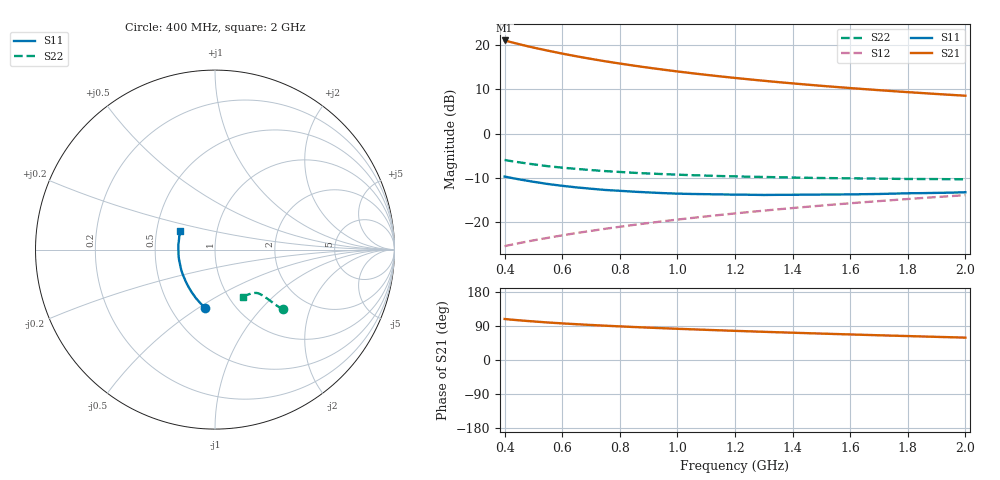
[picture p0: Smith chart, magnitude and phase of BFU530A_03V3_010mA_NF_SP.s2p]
! Filename:  P:\Prog\Test\Noise\ATS_data\Testdata_Net\06 Compressed Noise after Statistics\BFU530A_APG2013_33_A05_03p3V_010mA_NF_CM01_D.sf
! Date/Time: Tue 16/Apr/2013 15:10:58
! BFU530A_APG2013_33_A05_03p3V_1to25mA_NF_CM01_Bias5_R.sf
! Noise Parameter Data File
! BFU530A_APG2013_33_A05_03p3V_1to25mA_NF_CM01
! Date/time: Fri Apr 12 14:21:19 2013
! VAR V_out= 3.300000
! VAR I_out= 10.010000
! VAR V_in= 0.838100
! VAR I_in= 0.109800
! Device data file deembeded for feedlines and parallel
! Original file: \06 Compressed Noise after Statistics\BFU530A_APG2013_33_A05_03p3V_010mA_NF_CM01_R.sf
! Feed-files: PR017V01_150413_Feed1.s2p, PR017V01_150413_Feed2.s2p
! Parallel-file: PR017V01_150413_Par.s2p
# MHz S MA R 50
!  Freq-MHz  S11-mag  S11-arg  S21-mag  S21-arg  S12-mag  S12-arg  S22-mag  S22-arg
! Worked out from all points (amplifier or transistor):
!   37 points, 400 MHz to 2 GHz, reference 50 ohm
!   highest |S21| = 21.0 dB at 400 MHz (marker M1)
!   |S21| within 3 dB of that: start of sweep to 602.7 MHz
!   unconditionally stable (mu >= 1): 1.258 GHz to end of sweep
!   at 500 MHz: K = 0.81, MSG = 21.8 dB, |S12| = -24.1 dB
!   at 1.1 GHz: K = 0.99, MSG = 16.0 dB, |S12| = -18.7 dB
!   at 2 GHz: K = 1.01, MAG = 10.7 dB, |S12| = -13.9 dB
!   lowest NFmin = 0.79 dB at 433 MHz
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400  0.3283 -99.7  11.28 108.2  0.0538 64.5  0.5051 -41.3
420  0.3191 -102.5  10.85 106.7  0.05557 64.6  0.4923 -41.6
440  0.3097 -105.2  10.44 105.4  0.05731 64.7  0.481 -41.8
460  0.3016 -107.7  10.06 104.1  0.05907 64.8  0.4707 -42.1
500  0.2867 -112.7  9.376 101.8  0.06254 65.1  0.4513 -42.4
550  0.2708 -118.6  8.655 99.0  0.06678 65.5  0.4298 -42.7
600  0.2581 -123.9  8.015 96.6  0.07124 65.8  0.4138 -42.9
650  0.2478 -128.8  7.466 94.5  0.07567 66.1  0.4004 -43.2
700  0.2393 -133.6  6.987 92.4  0.08006 66.4  0.3886 -43.4
750  0.2317 -138.2  6.561 90.5  0.08456 66.7  0.3782 -43.5
800  0.2268 -142.5  6.19 88.7  0.08905 66.9  0.3701 -43.8
850  0.2215 -146.8  5.856 87.0  0.0936 67.1  0.3619 -44.2
900  0.2174 -150.8  5.556 85.4  0.09815 67.2  0.3554 -44.4
950  0.2136 -154.5  5.286 83.9  0.1027 67.3  0.35 -44.8
1050  0.2089 -161.6  4.817 81.0  0.1119 67.5  0.3403 -45.5
1150  0.2065 -168.2  4.429 78.2  0.1213 67.4  0.3326 -46.5
1200  0.2052 -171.1  4.259 76.9  0.126 67.4  0.3299 -47.0
1350  0.2042 -179.6  3.821 73.2  0.1401 67.0  0.3226 -48.8
1500  0.2058 172.5  3.47 69.7  0.1544 66.6  0.3161 -50.8
1600  0.2065 168.0  3.274 67.5  0.164 66.2  0.3137 -52.3
1750  0.2107 161.4  3.019 64.2  0.1783 65.4  0.3097 -54.6
2000  0.2185 152.0  2.682 59.0  0.2025 64.0  0.3061 -59.0
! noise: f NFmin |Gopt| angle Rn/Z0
400  0.8035  0.05764  179.6  0.0911
460  0.7976  0.0691  179.2  0.0813
600  0.8628  0.05575  -175.2  0.1001
800  0.8459  0.1263  -174.9  0.0754
1000  0.8506  0.1237  -169.6  0.0806
1200  0.9051  0.1474  -165.2  0.08
1400  0.9361  0.1818  -164.3  0.0752
1600  0.9405  0.2035  -154.8  0.0761
1800  0.9454  0.2305  -157.1  0.069
2000  0.9596  0.2466  -149.1  0.0781
